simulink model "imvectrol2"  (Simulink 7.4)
settings: Solver=ode45  StartTime=0.0  StopTime=12  MaxStep=2e-3  RelTol=1e-3

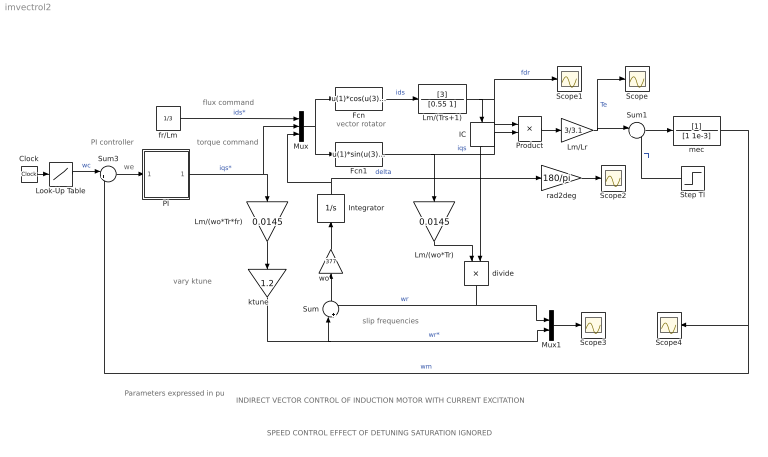
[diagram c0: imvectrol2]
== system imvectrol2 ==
  note: we
  note: PI controller
  note: Parameters expressed in pu
  note: vary ktune
  note: | |
  note: slip frequencies
  note: SPEED CONTROL EFFECT OF DETUNING SATURATION IGNORED
  note: INDIRECT VECTOR CONTROL OF INDUCTION MOTOR WITH CURRENT EXCITATION
  note: flux command
  note: vector rotator
  note: torque command
  Clock : Clock
  Fcn : Fcn  Expr=u(1)*cos(u(3))-u(2)*sin(u(3))
  Fcn1 : Fcn  Expr=u(1)*sin(u(3))+u(2)*cos(u(3))
  IC : InitialCondition  Value=.01
  Integrator : Integrator
  Lm/(Trs+1) : TransferFcn  Numerator=[3]  Denominator=[0.55 1]
  Lm/(wo*Tr) : Gain  Gain=0.0145  ParameterDataType=sfix(16)  ParameterScaling=2^0  OutDataType=sfix(16)  OutScaling=2^0
  Lm/(wo*Tr*fr) : Gain  Gain=0.0145  ParameterDataType=sfix(16)  ParameterScaling=2^0  OutDataType=sfix(16)  OutScaling=2^0
  Lm/Lr : Gain  Gain=3/3.1  ParameterDataType=sfix(16)  ParameterScaling=2^0  OutDataType=sfix(16)  OutScaling=2^0
  Look-Up Table : Lookup  InputValues=[0 3 3 6 6 10]  Table="[0 0 1 1 0.4  0.4]"  OutDataType=sfix(16)  OutScaling=2^0
  Mux : Mux  Inputs=3
  Mux1 : Mux  Inputs=2
  PI : Subsystem
  Product : Product  OutDataType=sfix(16)  OutScaling=2^0
  Scope{,1..4} (5 alike) : Scope
  Step Tl : Step  Time=9  SampleTime=0
  Sum : Sum  Inputs=|+-  OutDataType=sfix(16)  OutScaling=2^0
  Sum1 : Sum  Inputs=|+-  OutDataType=sfix(16)  OutScaling=2^0
  Sum3 : Sum  Inputs=|+-  OutDataType=sfix(16)  OutScaling=2^0
  divide : Product  Inputs=*/  OutDataType=sfix(16)  OutScaling=2^0
  fr/Lm : Constant  Value=1/3  OutDataType=sfix(16)  OutScaling=2^0
  ktune : Gain  Gain=1.2  ParameterDataType=sfix(16)  ParameterScaling=2^0  OutDataType=sfix(16)  OutScaling=2^0
  mec : TransferFcn  Denominator=[1 1e-3]
  rad2deg : Gain  Gain=180/pi  ParameterDataType=sfix(16)  ParameterScaling=2^0  OutDataType=sfix(16)  OutScaling=2^0
  wo : Gain  Gain=377  ParameterDataType=sfix(16)  ParameterScaling=2^0  OutDataType=sfix(16)  OutScaling=2^0
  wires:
  Mux/1 -> Fcn/1, Fcn1/1
  fr/Lm/1 -> Mux/1  "ids*"
  Fcn/1 -> Lm/(Trs+1)/1  "ids"
  wo/1 -> Integrator/1
  Product/1 -> Lm/Lr/1
  Lm/(Trs+1)/1 -> IC/1, Product/1, Scope1/1  "fdr"
  Fcn1/1 -> Product/2, Lm/(wo*Tr)/1  "iqs"
  IC/1 -> divide/2
  Lm/(wo*Tr)/1 -> divide/1
  divide/1 -> Sum/2, Mux1/1  "wr"
  Integrator/1 -> Mux/3, rad2deg/1  "delta"
  rad2deg/1 -> Scope2/1
  Lm/(wo*Tr*fr)/1 -> ktune/1
  ktune/1 -> Mux1/2, Sum/1  "wr*"
  Mux1/1 -> Scope3/1
  Sum/1 -> wo/1
  Sum1/1 -> mec/1
  Lm/Lr/1 -> Sum1/1, Scope/1  "Te"
  Step Tl/1 -> Sum1/2  "Tl"
  Sum3/1 -> PI/1(we)
  PI/1(wr) -> Mux/2, Lm/(wo*Tr*fr)/1  "iqs*"
  Look-Up Table/1 -> Sum3/1  "wc"
  Clock/1 -> Look-Up Table/1
  mec/1 -> Sum3/2, Scope4/1  "wm"

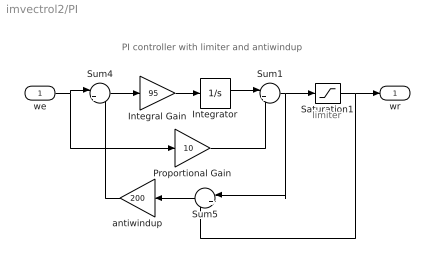
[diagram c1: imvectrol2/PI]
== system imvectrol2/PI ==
  note: limiter
  note: PI controller with limiter and antiwindup
  we : Inport  OutDataType=sfix(16)  OutScaling=2^0
  Integral Gain : Gain  Gain=95  ParameterDataType=sfix(16)  ParameterScaling=2^0  OutDataType=sfix(16)  OutScaling=2^0
  Integrator : Integrator
  Proportional Gain : Gain  Gain=10  ParameterDataType=sfix(16)  ParameterScaling=2^0  OutDataType=sfix(16)  OutScaling=2^0
  Saturation1 : Saturate  UpperLimit=2.5  LowerLimit=-1
  Sum1 : Sum  Inputs=|++  OutDataType=sfix(16)  OutScaling=2^0
  Sum4 : Sum  Inputs=|+-  OutDataType=sfix(16)  OutScaling=2^0
  Sum5 : Sum  Inputs=|+-  OutDataType=sfix(16)  OutScaling=2^0
  antiwindup : Gain  Gain=200  ParameterDataType=sfix(16)  ParameterScaling=2^0  OutDataType=sfix(16)  OutScaling=2^0
  wr : Outport
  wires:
  Integral Gain/1 -> Integrator/1
  Integrator/1 -> Sum1/1
  Proportional Gain/1 -> Sum1/2
  we/1 -> Sum4/1, Proportional Gain/1
  Sum4/1 -> Integral Gain/1
  Sum1/1 -> Saturation1/1, Sum5/1
  Sum5/1 -> antiwindup/1
  antiwindup/1 -> Sum4/2
  Saturation1/1 -> wr/1, Sum5/2
